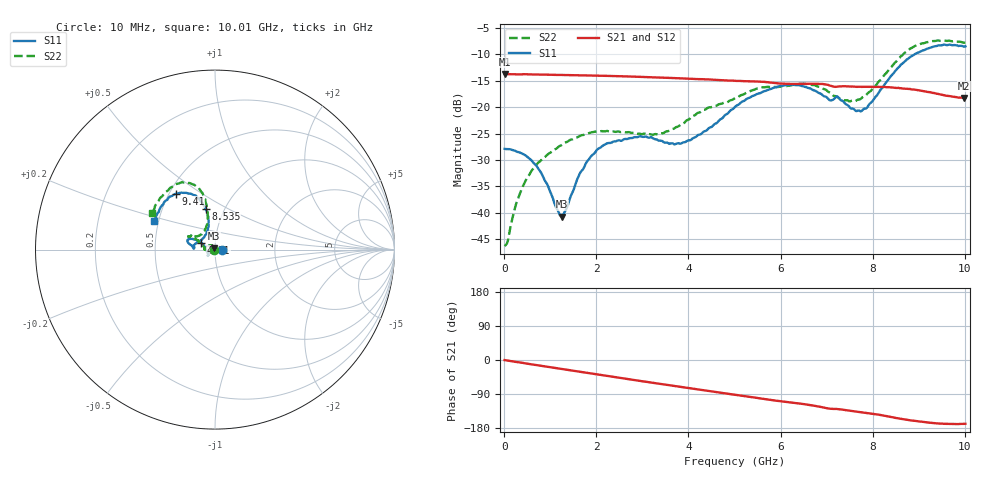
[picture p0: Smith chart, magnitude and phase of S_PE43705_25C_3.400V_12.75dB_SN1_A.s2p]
! Device ID: PE43705
! Serial: 1
! Insertion: A
! Impedance: 50 ohm
! Temp: 25C
! VDD: 3.400V
! Attenuation Step: 12.75dB
#  Hz  S  RI  R  50
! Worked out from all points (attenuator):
!   401 points, 10 MHz to 10.01 GHz, reference 50 ohm
!   highest |S21| = -13.76 dB at 10 MHz (marker M1); lowest = -18.3 dB at 9.985 GHz (marker M2)
!   lowest |S11| = -40.7 dB at 1.26 GHz (marker M3), VSWR 1.02, Z = 49.6 + j0.806 ohm
!   |S11| at or under -10 dB: start of sweep to 8.915 GHz
!   |S22| runs from -46.3 to -7.4 dB; largest |S21 - S12| = 0.0018
!   S11 on the Smith chart (normalised r, x): 10 MHz: 1.08, +0.00; 4.81 GHz: 0.86, +0.06; 8.535 GHz: 0.82, +0.39; 9.41 GHz: 0.54, +0.39; 10.01 GHz: 0.47, +0.17
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1e7  0.0403 0.000137  0.205 -0.00096  0.2052 -0.000815  -0.00484 0.000428
2.85e8  0.037 0.00748  0.2027 -0.0197  0.2027 -0.0196  -0.00584 0.0118
4.85e8  0.0319 0.0127  0.2009 -0.0333  0.201 -0.0331  -0.00962 0.0187
7.85e8  0.0192 0.0154  0.1956 -0.0525  0.1956 -0.0522  -0.0193 0.0241
1.26e9  -0.00438 0.00813  0.1836 -0.0812  0.1837 -0.0811  -0.0379 0.0225
1.685e9  -0.0245 -0.00555  0.1694 -0.1048  0.1694 -0.1047  -0.0523 0.0145
2.21e9  -0.0373 -0.0248  0.1475 -0.1304  0.1476 -0.1303  -0.0592 0.00294
2.935e9  -0.0402 -0.0343  0.1111 -0.1578  0.1114 -0.1578  -0.056 0.00296
3.36e9  -0.0383 -0.0292  0.0876 -0.1686  0.0878 -0.1684  -0.0551 0.00676
3.885e9  -0.0457 -0.00745  0.0575 -0.177  0.0578 -0.1768  -0.0666 0.0211
4.81e9  -0.0763 0.0376  0.00522 -0.1786  0.00562 -0.1783  -0.0979 0.0516
5.01e9  -0.0885 0.0472  -0.0053 -0.1771  -0.0051 -0.177  -0.1066 0.0581
5.985e9  -0.1466 0.0585  -0.0529 -0.1581  -0.0523 -0.1583  -0.1358 0.0752
6.685e9  -0.1429 0.0311  -0.0824 -0.1436  -0.0824 -0.1436  -0.1441 0.0726
7.335e9  -0.1104 0.0324  -0.1027 -0.1187  -0.1024 -0.119  -0.0907 0.0777
7.71e9  -0.0665 0.0645  -0.1142 -0.1058  -0.1137 -0.1058  -0.0607 0.1011
8.36e9  -0.0375 0.1836  -0.1326 -0.0781  -0.1321 -0.0787  -0.0434 0.2245
8.535e9  -0.0529 0.2252  -0.1355 -0.0675  -0.1347 -0.0688  -0.0545 0.2716
8.935e9  -0.1075 0.3014  -0.1374 -0.0474  -0.1371 -0.0466  -0.1177 0.362
9.41e9  -0.2189 0.3108  -0.1301 -0.029  -0.1296 -0.029  -0.2182 0.3649
9.985e9  -0.3319 0.1653  -0.1196 -0.0247  -0.12 -0.0249  -0.3437 0.2135
1.001e10  -0.3395 0.1567  -0.1199 -0.0248  -0.1204 -0.0253  -0.3514 0.2027
